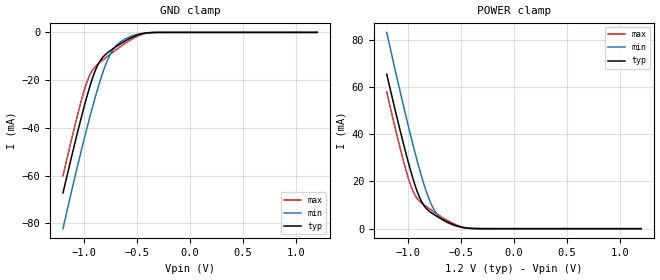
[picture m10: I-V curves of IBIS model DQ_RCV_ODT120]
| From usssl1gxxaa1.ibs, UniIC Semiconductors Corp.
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|   Model DQ_RCV_ODT120
[Model] DQ_RCV_ODT120
Model_type Input
Vinl =  0.500V
Vinh =  0.700V
C_comp   1.373pF   1.353pF   1.403pF
[Model Spec]
Vinh   0.700V   0.670V   0.750V
Vinl   0.500V   0.470V   0.550V
[Add Submodel]
|  Submodel_name   Mode
DQ_ODT120   Non-Driving
[Temperature Range]   25.000   0.125k   -40.000
[Voltage Range]   1.200V   1.140V   1.300V
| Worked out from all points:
|   GND clamp passes 1 mA (typ) near -0.49 V on its own axis
|   POWER clamp passes 1 mA (typ) near -0.53 V on its own axis
[GND_clamp]
|Voltage   I(typ)   I(min)   I(max)
-1.2V     -67.26mA   -82.22mA   -60.1mA
-1.05V    -39.62mA   -53.62mA   -32.4mA
-1V       -31.05mA   -44.64mA   -24.37mA
-950mV    -23.16mA   -36.01mA   -18.1mA
-925mV    -19.62mA   -31.85mA   -16.02mA
-875mV    -13.89mA   -23.97mA   -13.48mA
-800mV    -9.288mA   -13.81mA   -10.72mA
-750mV    -7.535mA   -8.829mA   -8.993mA
-675mV    -5.274mA   -4.578mA   -6.506mA
-525mV    -1.587mA   -1.138mA   -2.208mA
-375mV    -90.13uA   -87.27uA   -132.9uA
1.2V      0A         0A         0A
[POWER_clamp]
|Voltage   I(typ)   I(min)   I(max)
-1.2V     65.51mA    83.21mA    57.91mA
-1.05V    37.38mA    53.57mA    29.99mA
-1V       28.74mA    44.18mA    21.95mA
-950mV    20.85mA    35.16mA    15.65mA
-925mV    17.34mA    30.84mA    13.56mA
-875mV    11.74mA    22.7mA     11.06mA
-800mV    7.436mA    12.47mA    8.502mA
-750mV    5.864mA    7.69mA     6.933mA
-675mV    3.901mA    3.837mA    4.735mA
-525mV    971.5uA    903.1uA    1.25mA
-400mV    85.95uA    125.9uA    91.19uA
1.2V      0A         0A         0A
